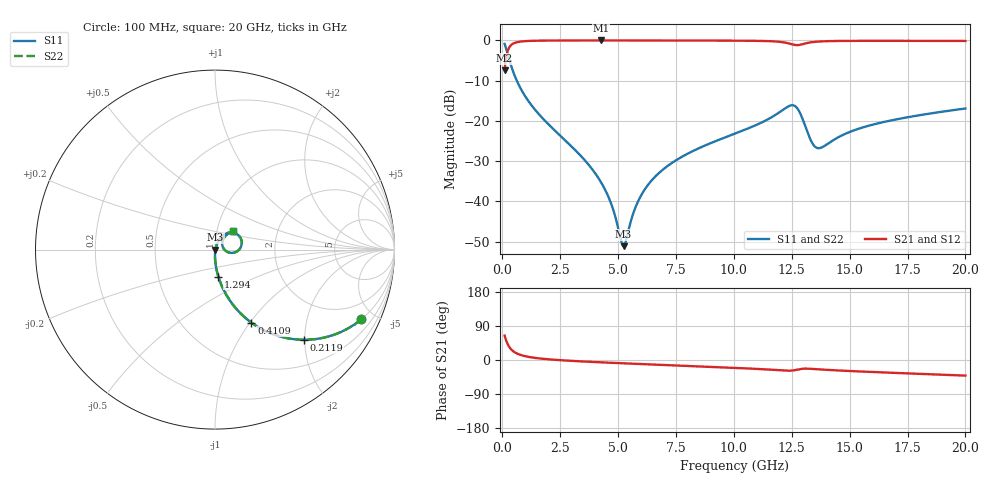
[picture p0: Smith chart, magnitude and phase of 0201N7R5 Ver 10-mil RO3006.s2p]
# GHz S MA R 50
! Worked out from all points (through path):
!   1601 points, 100 MHz to 20 GHz, reference 50 ohm
!   highest |S21| = -0.02 dB at 4.267 GHz (marker M1); lowest = -7.4 dB at 100 MHz (marker M2)
!   group delay of S21, straight-line fit = 7.18 ps
!   lowest |S11| = -51.1 dB at 5.237 GHz (marker M3), VSWR 1.01, Z = 50.3 - j0.0445 ohm
!   |S11| at or under -10 dB: 625.6 MHz to end of sweep
!   |S22| runs from -51.1 to -0.9 dB; largest |S21 - S12| = 0
!   S11 on the Smith chart (normalised r, x): 100 MHz: 0.99, -4.21; 211.9 MHz: 0.99, -1.98; 410.9 MHz: 0.99, -1.02; 1.294 GHz: 0.99, -0.31; 20 GHz: 1.19, +0.25
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0.1  0.9039 -25.5  0.4272 64.5  0.4272 64.5  0.9039 -25.5
0.2119375  0.7057 -45.4  0.7077 44.5  0.7077 44.5  0.7057 -45.4
0.4109375  0.4554 -63.5  0.8893 26.4  0.8893 26.4  0.4554 -63.5
0.7094375  0.281 -74.7  0.9586 15.1  0.9586 15.1  0.281 -74.7
1.294  0.1519 -82.9  0.987 6.6  0.987 6.6  0.1519 -82.9
3.420812  0.03599 -90.2  0.997 -3.7  0.997 -3.7  0.03599 -90.2
4.266563  0.01724 -87.9  0.9973 -6.2  0.9973 -6.2  0.01724 -87.9
4.701875  0.009354 -81.1  0.9972 -7.4  0.9972 -7.4  0.009354 -81.1
5.137187  0.003192 -39.0  0.9971 -8.5  0.9971 -8.5  0.003192 -39.0
5.236688  0.00278 -9.2  0.9971 -8.8  0.9971 -8.8  0.00278 -9.2
5.908313  0.01064 63.2  0.9968 -10.5  0.9968 -10.5  0.01064 63.2
6.741625  0.0222 69.0  0.9963 -12.6  0.9963 -12.6  0.0222 69.0
7.997813  0.03905 68.9  0.9953 -15.6  0.9953 -15.6  0.03905 68.9
10.05  0.06955 64.4  0.9916 -20.8  0.9916 -20.8  0.06955 64.4
11.61712  0.1104 54.8  0.9754 -25.7  0.9754 -25.7  0.1104 54.8
12.5375  0.1564 21.3  0.8901 -27.7  0.8901 -27.7  0.1564 21.3
12.836  0.1291 -2.4  0.8786 -24.1  0.8786 -24.1  0.1291 -2.4
13.37081  0.05398 -1.8  0.9493 -23.4  0.9493 -23.4  0.05398 -1.8
13.74394  0.04619 26.1  0.97 -25.0  0.97 -25.0  0.04619 26.1
15.03744  0.07351 51.9  0.9855 -29.2  0.9855 -29.2  0.07351 51.9
16.69162  0.09995 52.0  0.9866 -33.4  0.9866 -33.4  0.09995 52.0
20  0.1426 46.0  0.9824 -41.2  0.9824 -41.2  0.1426 46.0
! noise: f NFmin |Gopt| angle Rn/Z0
0.1  0.0007  0.9387  0.4119  0.00255
2.301  0.004057  0.7762  4.011  0.003703
4.515  0.006764  0.742  7.622  0.005234
6.729  0.009303  0.7238  11.23  0.006623
8.943  0.01239  0.725  14.82  0.008807
11.14  0.02187  0.7982  18.48  0.02186
13.36  0.05255  0.8943  22.25  0.1044
15.57  0.02433  0.7547  25.68  0.01907
17.79  0.02263  0.7081  29.05  0.01432
20  0.02336  0.6875  32.41  0.01343
